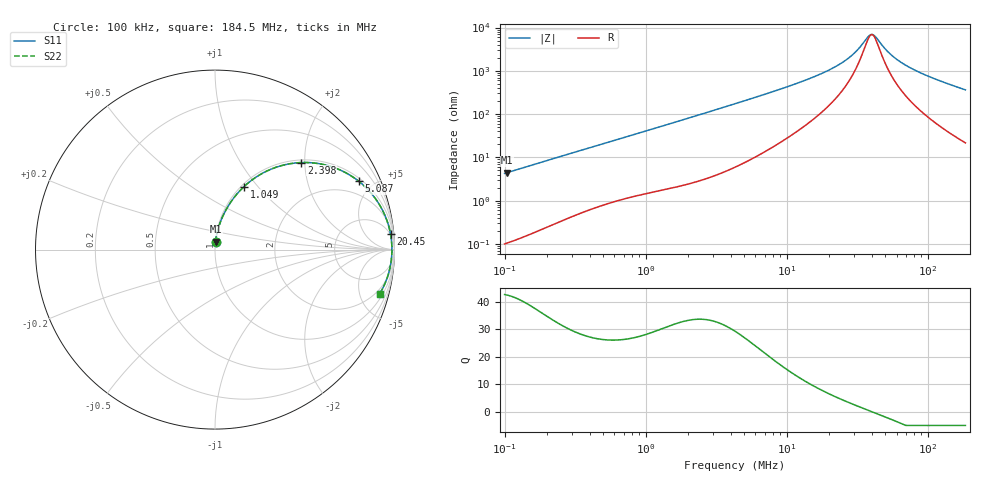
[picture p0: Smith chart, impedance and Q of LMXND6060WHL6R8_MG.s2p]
! LMXND6060WHL6R8_MG  S-PARAMETER MODEL  ( General Type )
! Model Generated by TAIYO YUDEN Corporation (https://www.yuden.co.jp/en/)
! Version 1.0
! TAIYO YUDEN Control No. 191025NI43SB-FBB
! Copyright(c) 2019 TAIYO YUDEN CO.,LTD. All Rights Reserved.
! Product Description (link to TY-COMPAS)
! https://ds.yuden.co.jp/TYCOMPAS/or/detail?pn=LMXND6060WHL6R8MMG&u=M
! Products Name : Inductors
! Characteristics :
!  Inductance : 6.8 uH , SRF(min) : 25 MHz , DC Resistance(max) : 0.0559 Ohm
!  Rated Current : Saturation :2600 mA , Temp Rise : 2500 mA (40 degC)
!  Case Size : 6.0 x 6.0 / 0.236 x 0.236 [mm/inch] , Thickness : 2.8 / 0.11 [mm/inch]
!  (Conditions: Temperature = 25 degC , DC Bias Current/Voltage = 0A / 0V)
! External Node Assignments :
!  1  o---GGG---o  2
! GND o---------o GND
! Frequency Range : 0.1MHz  -  184.468258MHz  [ 402 STEP ]
# MHz S RI R 50
! Freq[MHz].  S11 Real  S11 Imag  S21 Real  S21 Imag  S12 Real  S12 Imag  S22 Real  S22 Imag
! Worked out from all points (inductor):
!   401 points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, 100 kHz to 184.5 MHz, reference 50 ohm
!   read as one part in series: L = 6.77 uH near 103.8 kHz
!   highest Q = 42.4 at 103.8 kHz (marker M1), where L = 6.78 uH
!   self-resonance near 39.48 MHz
!   S11 on the Smith chart (normalised r, x): 100 kHz: 1.00, +0.09; 1.049 MHz: 1.03, +0.85; 2.398 MHz: 1.06, +1.92; 5.087 MHz: 1.15, +4.12; 20.45 MHz: 4, +21; 184.5 MHz: 1.43, -7.25
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0.1  0.00281 0.0424  0.9972 -0.0424  0.9972 -0.0424  0.00281 0.0424
0.103832  0.00299 0.0441  0.997 -0.0441  0.997 -0.0441  0.00299 0.0441
0.352405  0.0261 0.1427  0.9739 -0.1427  0.9739 -0.1427  0.0261 0.1427
0.655361  0.0756 0.2459  0.9244 -0.2459  0.9244 -0.2459  0.0756 0.2459
1.048577  0.1615 0.3508  0.8385 -0.3508  0.8385 -0.3508  0.1615 0.3508
1.241892  0.2088 0.39  0.7912 -0.39  0.7912 -0.39  0.2088 0.39
2.398015  0.4816 0.485  0.5184 -0.485  0.5184 -0.485  0.4816 0.485
4.294977  0.7431 0.4202  0.2569 -0.4202  0.2569 -0.4202  0.7431 0.4202
5.086793  0.8006 0.3812  0.1994 -0.3812  0.1994 -0.3812  0.8006 0.3812
8.29333  0.9106 0.2595  0.0894 -0.2595  0.0894 -0.2595  0.9106 0.2595
15.13571  0.9665 0.1353  0.0335 -0.1353  0.0335 -0.1353  0.9665 0.1353
20.44747  0.9778 0.0874  0.0222 -0.0874  0.0222 -0.0874  0.9778 0.0874
28.68178  0.984 0.0413  0.016 -0.0413  0.016 -0.0413  0.984 0.0413
32.10664  0.985 0.0271  0.015 -0.0271  0.015 -0.0271  0.985 0.0271
37.31757  0.9857 0.00863  0.0143 -0.00863  0.0143 -0.00863  0.9857 0.00863
39.48278  0.9858 0.00175  0.0142 -0.00175  0.0142 -0.00175  0.9858 0.00175
42.5664  0.9857 -0.0074  0.0143 0.0074  0.0143 0.0074  0.9857 -0.0074
53.33896  0.9844 -0.0353  0.0156 0.0353  0.0156 0.0353  0.9844 -0.0353
64.37135  0.982 -0.0597  0.018 0.0597  0.018 0.0597  0.982 -0.0597
83.7529  0.9758 -0.0971  0.0242 0.0971  0.0242 0.0971  0.9758 -0.0971
121.9821  0.9581 -0.1606  0.0419 0.1606  0.0419 0.1606  0.9581 -0.1606
184.4683  0.9168 -0.2479  0.0832 0.2479  0.0832 0.2479  0.9168 -0.2479
